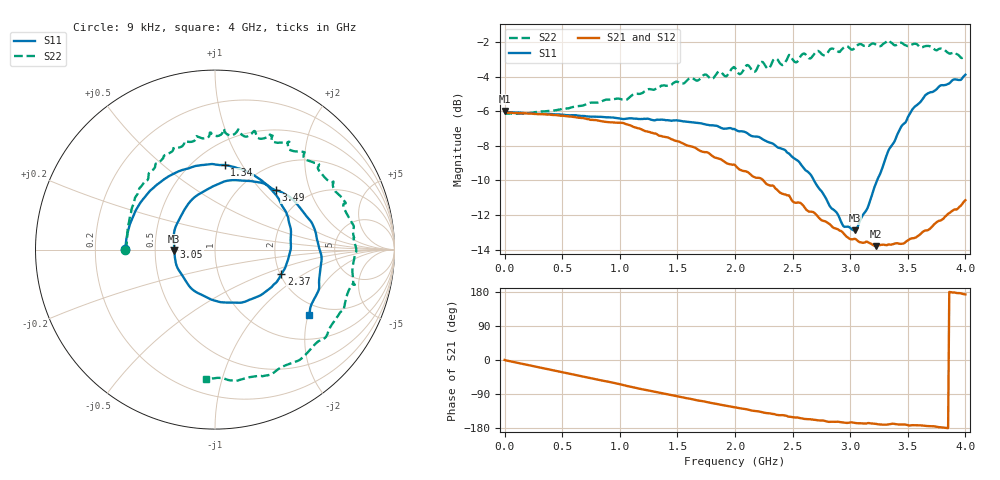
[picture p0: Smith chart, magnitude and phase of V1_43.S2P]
! ZVRE, 3.40
! symbol freq-unit parameter-type data-format keyword impedance-ohm
#  HZ  S  RI  R  50
! freq  reS11  imS11  reS21  imS21  reS12  imS12  reS22  imS22
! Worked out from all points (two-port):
!   401 points, 9 kHz to 4 GHz, reference 50 ohm
!   highest |S21| = -5.98 dB at 9 kHz (marker M1); lowest = -13.8 dB at 3.22 GHz (marker M2)
!   |S21| within 3 dB of the highest: start of sweep to 1.921 GHz
!   lowest |S11| = -12.9 dB at 3.04 GHz (marker M3), VSWR 1.59, Z = 31.5 - j0.51 ohm
!   |S11| at or under -10 dB: 2.685 GHz to 3.233 GHz (548.1 MHz wide, 18.5 % of centre)
!   |S22| runs from -6.1 to -1.9 dB; largest |S21 - S12| = 0.01
!   S11 on the Smith chart (normalised r, x): 9 kHz: 0.33, +0.00; 1.34 GHz: 0.70, +0.84; 2.37 GHz: 2.03, -0.66; 3.05 GHz: 0.63, +0.02; 3.49 GHz: 1.42, +1.21; 4 GHz: 1.66, -2.04
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9000  -0.4999 0.00118  0.5021 0.00133  0.502 -0.00152  -0.5004 -0.000327
3.400082e8  -0.4529 0.193  0.456 -0.1839  0.4599 -0.1814  -0.4848 0.1256
6.700075e8  -0.339 0.3478  0.3495 -0.328  0.3554 -0.3251  -0.4544 0.2531
1.050007e9  -0.1376 0.4564  0.1745 -0.4263  0.1802 -0.428  -0.3753 0.3889
1.340006e9  0.0543 0.4705  0.0295 -0.4252  0.0329 -0.4279  -0.287 0.513
1.620005e9  0.2343 0.403  -0.089 -0.3864  -0.0848 -0.3888  -0.1694 0.6031
2.000004e9  0.4084 0.1753  -0.2008 -0.287  -0.197 -0.2905  0.0513 0.6681
2.200004e9  0.4227 0.0102  -0.229 -0.2261  -0.226 -0.2303  0.2029 0.6448
2.370004e9  0.3696 -0.1369  -0.243 -0.1693  -0.2395 -0.1754  0.319 0.6313
2.670003e9  0.1302 -0.2961  -0.2359 -0.1006  -0.2359 -0.1069  0.5255 0.4937
2.870003e9  -0.1126 -0.2318  -0.22 -0.0661  -0.2199 -0.0714  0.6588 0.3713
3.040002e9  -0.2264 -0.00767  -0.2079 -0.0518  -0.2083 -0.0553  0.7431 0.1836
3.050002e9  -0.2273 0.0126  -0.2076 -0.0501  -0.2091 -0.0522  0.7544 0.165
3.120002e9  -0.2188 0.1287  -0.2039 -0.0453  -0.2047 -0.0522  0.7681 0.1027
3.220002e9  -0.1256 0.2814  -0.1998 -0.0415  -0.2023 -0.0458  0.7818 -0.0238
3.300002e9  0.0072 0.3602  -0.203 -0.0335  -0.2053 -0.0375  0.7697 -0.1788
3.340001e9  0.0705 0.3841  -0.2028 -0.0379  -0.2063 -0.0384  0.7781 -0.1945
3.490001e9  0.3375 0.3302  -0.2084 -0.0327  -0.2122 -0.0317  0.6718 -0.3881
3.640001e9  0.5236 0.1696  -0.2241 -0.0256  -0.2273 -0.0256  0.5151 -0.5742
3.760001e9  0.5856 -0.00883  -0.2402 -0.0135  -0.2426 -0.013  0.3442 -0.672
3.9e9  0.5789 -0.2212  -0.2598 0.00836  -0.2596 0.0145  0.1249 -0.7301
4e9  0.5261 -0.3638  -0.2752 0.033  -0.2719 0.0371  -0.0513 -0.7226
